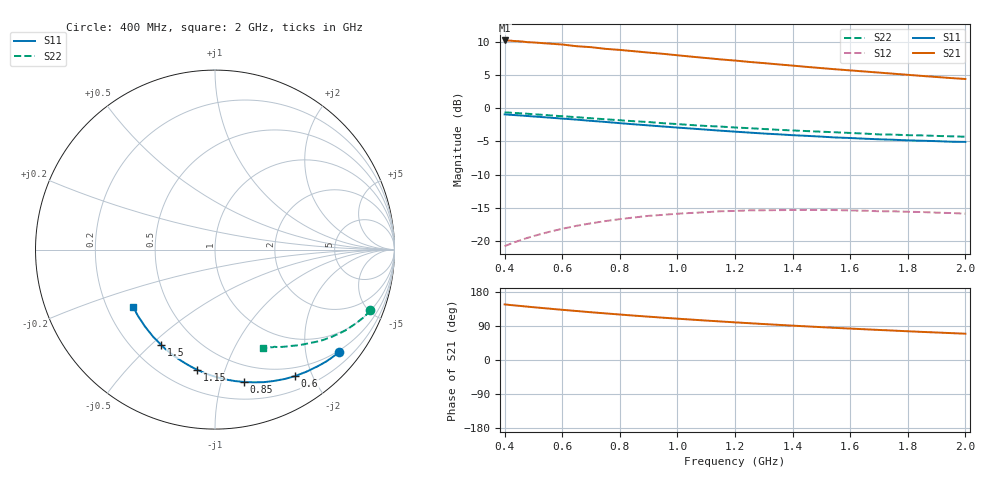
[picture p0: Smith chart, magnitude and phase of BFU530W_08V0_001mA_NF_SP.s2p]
! Filename:  P:\Prog\Test\Noise\ATS_data\Testdata_Net\06 Compressed Noise after Statistics\BFU530W_APM2013_09_A05_08p0V_001mA_NF_CM01_D.sf
! Date/Time: Tue 26/Mar/2013 18:06:04
! BFU530W_APM2013_09_A05_08p0V_1to25mA_NF_CM01_Bias1_R.sf
! Noise Parameter Data File
! BFU530W_APM2013_09_A05_08p0V_1to25mA_NF_CM01
! Date/time: Thu Mar 21 21:44:48 2013
! freq range =  0.4000 to  2.0000 GHz, 37 points
! bias range =  1.0000 to 25.0050 mA, 9 points
! bias supplies used: 1 1 0 0 0 0
! VAR bias_mode= 1  ! Specify V_out, I_out
! VAR bias_var = 1  ! Bias variable = I_out
! VAR V_out= 8.001000
! VAR I_out= 1.000000
! VAR V_in= 0.780800
! VAR I_in= 0.009801
! Device data file deembeded for feedlines and parallel
! Original file: \06 Compressed Noise after Statistics\BFU530W_APM2013_09_A05_08p0V_001mA_NF_CM01_R.sf
! Feed-files: PR019V01_070313_Feed1.s2p, PR019V01_070313_Feed2.s2p
! Parallel-file: PR019V01_070313_Par.s2p
# MHz S MA R 50
!  Freq-MHz  S11-mag  S11-arg  S21-mag  S21-arg  S12-mag  S12-arg  S22-mag  S22-arg
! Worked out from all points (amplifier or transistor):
!   37 points, 400 MHz to 2 GHz, reference 50 ohm
!   highest |S21| = 10.2 dB at 400 MHz (marker M1)
!   |S21| within 3 dB of that: start of sweep to 1.194 GHz
!   unconditionally stable (mu >= 1): nowhere
!   at 500 MHz: K = 0.20, MSG = 14.6 dB, |S12| = -19.2 dB
!   at 1.1 GHz: K = 0.40, MSG = 11.6 dB, |S12| = -15.6 dB
!   at 2 GHz: K = 0.76, MSG = 10.1 dB, |S12| = -15.9 dB
!   lowest NFmin = 0.41 dB at 420 MHz
!   S11 on the Smith chart (normalised r, x): 400 MHz: 0.46, -2.71; 600 MHz: 0.38, -1.76; 850 MHz: 0.34, -1.18; 1.15 GHz: 0.33, -0.81; 1.5 GHz: 0.32, -0.54; 2 GHz: 0.31, -0.29
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400  0.8969 -39.6  3.224 146.7  0.0917 64.7  0.9293 -21.3
420  0.8907 -41.5  3.214 145.1  0.09548 63.6  0.9238 -22.2
460  0.8787 -45.2  3.167 142.2  0.1026 61.5  0.9129 -24.1
480  0.8721 -46.9  3.128 140.8  0.106 60.4  0.9068 -24.9
500  0.8653 -48.8  3.116 139.3  0.1092 59.3  0.9 -25.8
600  0.8343 -57.6  3.006 132.5  0.1239 54.5  0.8687 -29.9
650  0.8192 -61.6  2.918 129.3  0.1305 52.3  0.855 -31.7
700  0.802 -65.9  2.87 126.0  0.1362 50.1  0.8391 -33.6
750  0.7872 -69.7  2.789 123.0  0.1416 48.2  0.8244 -35.2
800  0.7707 -73.7  2.737 120.0  0.1464 46.3  0.8107 -37.0
850  0.7555 -77.6  2.675 117.1  0.1507 44.4  0.7964 -38.5
950  0.7274 -84.9  2.558 111.7  0.1577 41.0  0.7702 -41.5
1050  0.7014 -91.8  2.434 106.5  0.163 38.1  0.7456 -44.1
1150  0.6766 -98.5  2.323 101.7  0.1678 35.4  0.7266 -46.5
1200  0.6654 -101.6  2.276 99.3  0.1686 34.2  0.7149 -47.9
1250  0.6544 -104.8  2.223 97.1  0.1704 33.0  0.7067 -48.9
1350  0.6354 -110.8  2.131 92.8  0.1711 31.1  0.687 -51.3
1500  0.6102 -119.5  1.998 86.7  0.1716 28.4  0.6647 -54.5
1600  0.5959 -125.1  1.921 82.9  0.1701 27.2  0.6505 -56.6
1750  0.5784 -132.9  1.813 77.6  0.1676 26.0  0.632 -59.4
1850  0.5684 -137.9  1.745 74.2  0.1655 25.3  0.6235 -61.3
2000  0.5571 -145.2  1.655 69.4  0.161 25.4  0.6094 -64.2
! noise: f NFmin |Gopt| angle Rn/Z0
400  0.4609  0.6942  24.7  0.3086
460  0.4665  0.6867  28.8  0.3315
600  0.522  0.6833  35.76  0.3334
800  0.6037  0.6513  48.85  0.281
1000  0.7675  0.6432  60.55  0.3044
1200  0.7752  0.6283  73.87  0.2635
1400  0.8025  0.5958  87.32  0.2115
1600  0.7601  0.5412  101.7  0.1513
1800  0.9423  0.6067  112.4  0.1402
2000  1.007  0.5628  122.5  0.1384
